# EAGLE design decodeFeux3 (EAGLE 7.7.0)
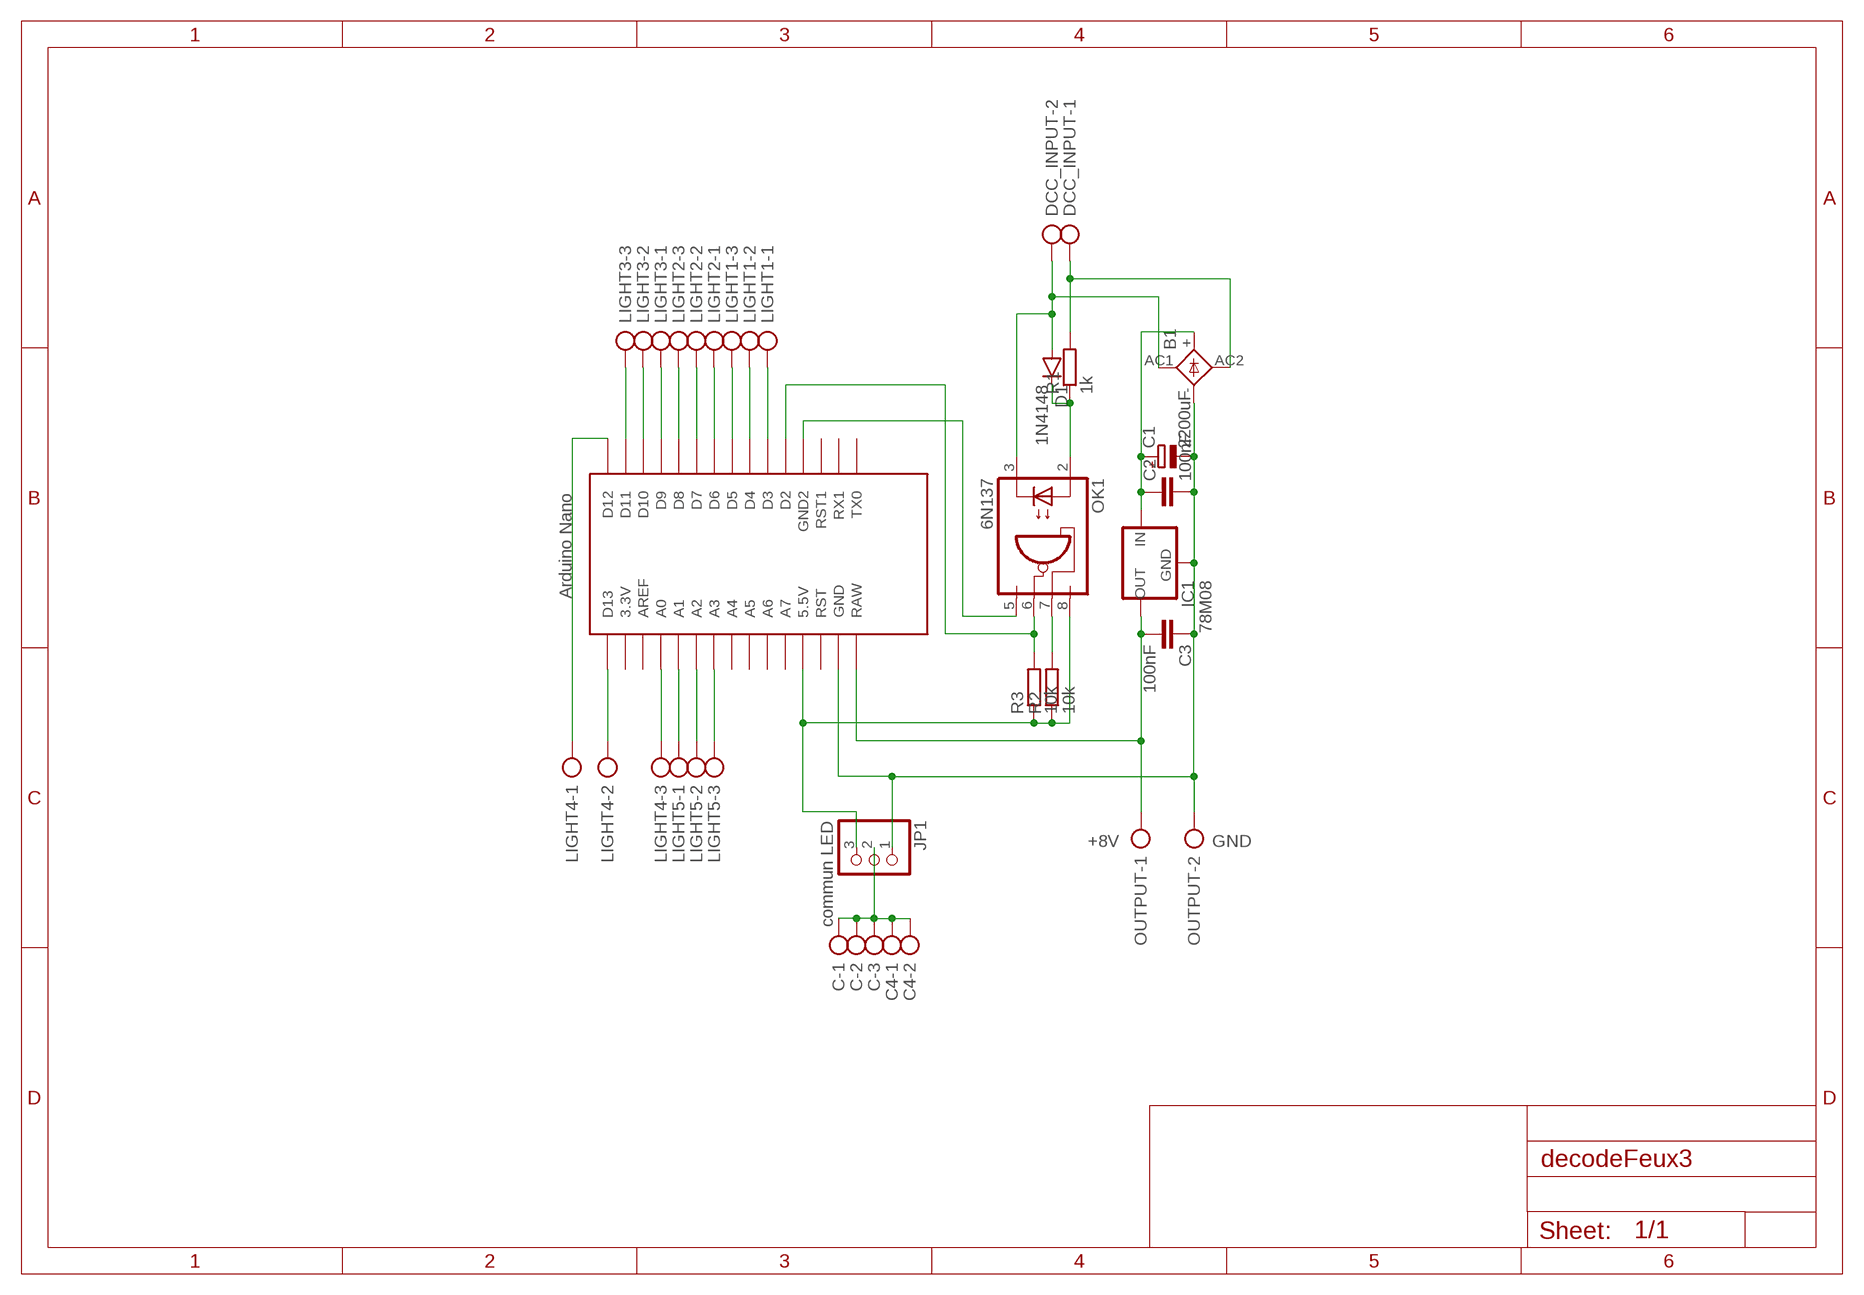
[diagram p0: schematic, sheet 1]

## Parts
B1  2KBP  [2KBP]
C  AK300/3  [AK300/3]
C1  2200uF  CPOL-EUE7.5-16  [E7,5-16]
C2  100nF  C-EU050-025X075  [C050-025X075]
C3  100nF  C-EU050-025X075  [C050-025X075]
C4  AK300/2  [AK300/2]
D1  1N4148  DIODE1N4148  [DIODE-1N4148]
DCC_INPUT  AK300/2  [AK300/2]
IC1  78M08  R-78C1.8-1.0  [SIP3]
JP1  commun LED  PINHD-1X3  [1X03]
LIGHT1  AK300/3  [AK300/3]
LIGHT2  AK300/3  [AK300/3]
LIGHT3  AK300/3  [AK300/3]
LIGHT4  AK300/3  [AK300/3]
LIGHT5  AK300/3  [AK300/3]
OK1  6N137  [DIL08]
OUTPUT  AK300/2  [AK300/2]
R1  1k  R-EU_0207/10  [0207/10]
R2  10k  R-EU_0207/10  [0207/10]
R3  10k  R-EU_0207/10  [0207/10]
U$1  NANO  [NANO]

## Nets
N$1: LIGHT4.1 U$1.D12
N$2: LIGHT3.3 U$1.D11
N$3: LIGHT3.2 U$1.D10
N$4: LIGHT3.1 U$1.D9
N$5: LIGHT2.3 U$1.D8
N$6: LIGHT2.2 U$1.D7
N$7: LIGHT2.1 U$1.D6
N$8: LIGHT1.3 U$1.D5
N$9: LIGHT1.2 U$1.D4
N$10: LIGHT1.1 U$1.D3
N$11: LIGHT4.2 U$1.D13
N$12: LIGHT4.3 U$1.A0
N$13: LIGHT5.1 U$1.A1
N$14: LIGHT5.2 U$1.A2
N$15: LIGHT5.3 U$1.A3
N$17: OK1.6(VO) R3.2 U$1.D2
N$18: OK1.7(VE) R2.2
N$19: JP1.3 OK1.8(VCC) R2.1 R3.1 U$1.5V(5.5V)
N$20: OK1.5(GND) U$1.GND1(GND2)
N$21: B1.AC2 DCC_INPUT.1 R1.2
N$22: B1.AC1 D1.A DCC_INPUT.2 OK1.3(C)
N$23: D1.C OK1.2(A) R1.1
N$24: B1.+ C1.+ C2.1 IC1.1(IN)
N$25: B1.- C1.- C2.2 C3.1 IC1.2(GND) JP1.1 OUTPUT.2 U$1.GND
N$26: C3.2 IC1.3(OUT) OUTPUT.1 U$1.RAW
N$28: C4.1 C4.2 C.1 C.2 C.3 JP1.2
Unconnected: U$1.3.3V U$1.A4 U$1.A5 U$1.A6 U$1.A7 U$1.AREF U$1.ICSP1 U$1.ICSP2 U$1.ICSP3 U$1.ICSP4 U$1.ICSP5 U$1.ICSP6 U$1.RST U$1.RST1 U$1.RX1 U$1.TX0

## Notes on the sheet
- +8V | GND

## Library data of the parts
B1 = rectifier:2KBP: RECTIFIER grid 3 x 3,81 mm
C LIGHT1-LIGHT5 = con-ptr500:AK300/3: CONNECTOR; OC_FARNELL: unknown; OC_NEWARK: unknown
C1 = resistor:CPOL-EU: POLARIZED CAPACITOR, European symbol
C2 C3 = rcl:C-EU: CAPACITOR, European symbol
C4 DCC_INPUT OUTPUT = con-ptr500:AK300/2: CONNECTOR; OC_FARNELL: unknown; OC_NEWARK: unknown
D1 = SparkFun-DiscreteSemi:DIODE: Diode; PROD_ID: DIO-08378
IC1 = r-78xx_10:R-78C*-1.0: Innoline R-78Cxx-1.0 Series Switching Regulators - 1.0A, Wide Input Range, High Efficiency Source: http://www.recom-international.com/pdf/Innoline/R-78Cxx-1.0.pdf; MF: Recom; MPN: R-78C1.8-1.0; OC_FARNELL: 1903038; OC_NEWARK: 62X9492
JP1 = adafruit:PINHD-1X3: PIN HEADER
OK1 = optocoupler:6N137: MOTOROLA OPTO COUPLER; MPN: 6N137; OC_FARNELL: 1328376; OC_NEWARK: 52M1895
R1-R3 = resistor:R-EU_: RESISTOR, European symbol
U$1 = Arduino-clone:NANO: Arduino Nano

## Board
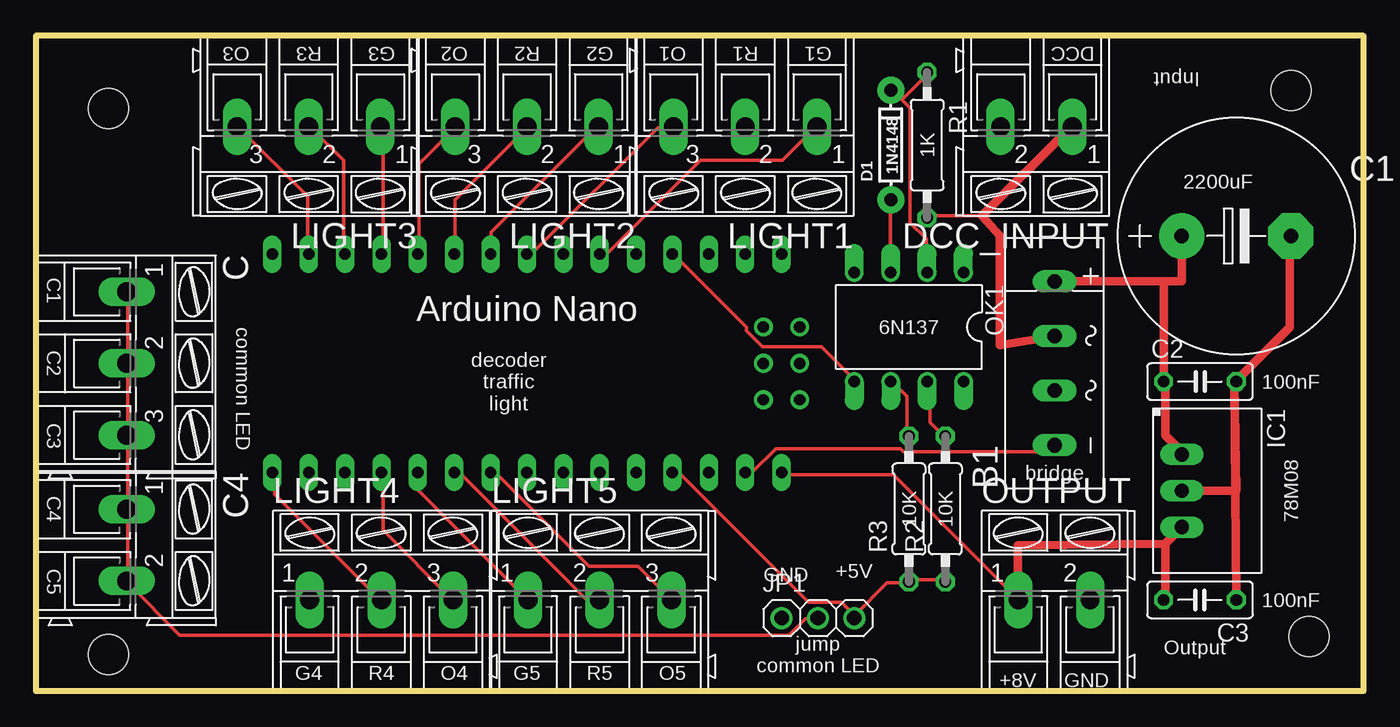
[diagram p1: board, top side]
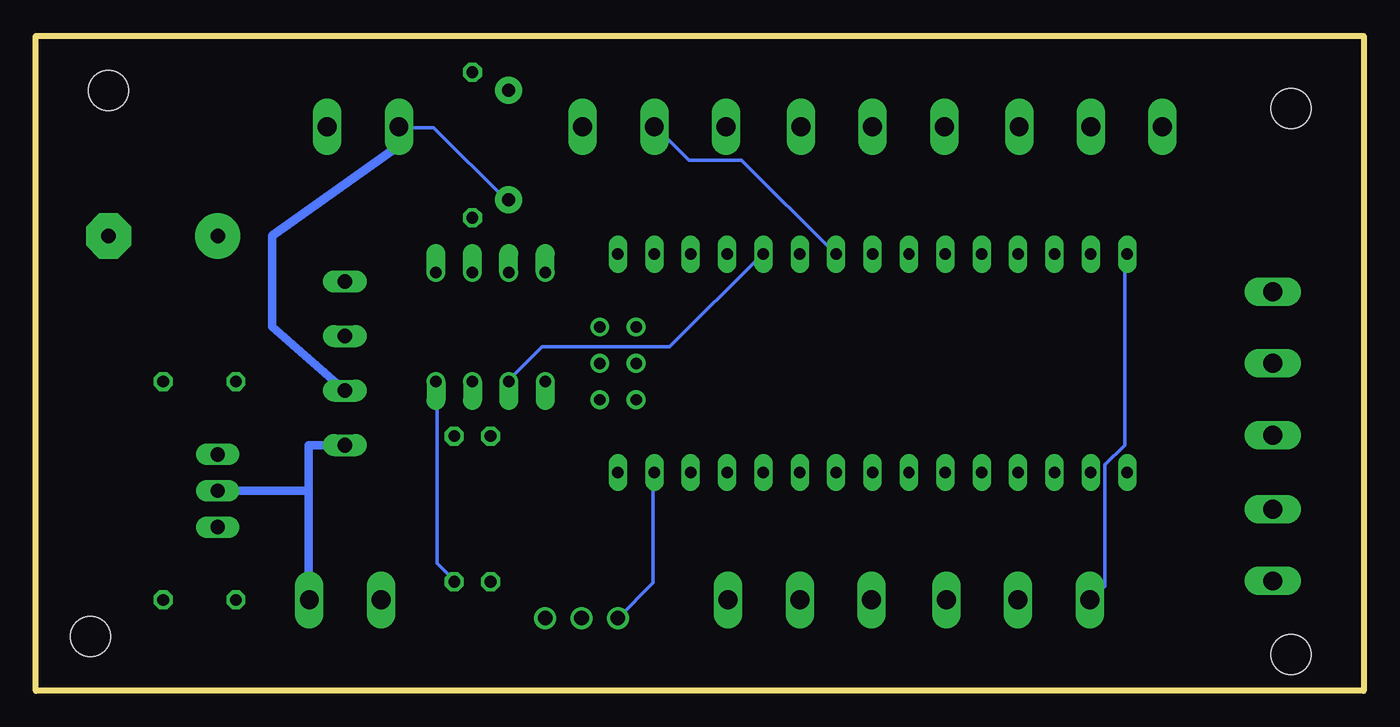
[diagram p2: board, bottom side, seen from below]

Size 92.71 x 45.72 mm. Coordinates in mm from the lower left corner, seen from the top.
Outline: 0,0 92.71,0 92.71,45.72 0,45.72 0,0
Copper layers (1*16): Top 0.035mm / dielectric 1.5mm / Bottom 0.035mm
Design rules "default": minimum track width 10mil, minimum drill 24mil, track to track 8mil, track to pad 8mil, pad to pad 8mil, via to via 8mil, smd to smd 8mil, copper to edge 40mil, drill to drill 8mil, minimum pad ring 10mil, minimum via ring 8mil, stop-mask expansion 4mil, vias tented up to drill 0mil, thermal gap 10mil
Holes 2.8 mm at 5.08,40.64 5.08,2.54 88.9,3.81 87.63,41.91

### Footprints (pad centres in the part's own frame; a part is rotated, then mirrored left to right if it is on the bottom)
2KBP = drill 1.016 long: + 5.715,0; - -5.715,0; AC1 -1.905,0; AC2 1.905,0
AK300/3 = drill 1.321 long: 1 -5.004,0; 2 0,0; 3 5.004,0
E7,5-16 = drill 1.016 pad 3.15: + -3.81,0 | drill 1.016 pad 3.15 octagon: - 3.81,0
C050-025X075 = drill 0.813 octagon: 1 -2.54,0; 2 2.54,0
AK300/2 = drill 1.321 long: 1 -2.515,0; 2 2.489,0
DIODE-1N4148 = drill 0.9 pad 1.88: A -3.81,0; C 3.81,0
SIP3 = drill 1 long: 1 -2.54,0; 2 0,0; 3 2.54,0
1X03 = drill 1.016: 1 -2.54,0; 2 0,0; 3 2.54,0
DIL08 = drill 0.813 offset: 1 -3.81,-3.81; 2 -1.27,-3.81; 3 1.27,-3.81; 4 3.81,-3.81; 5 3.81,3.81; 6 1.27,3.81; 7 -1.27,3.81; 8 -3.81,3.81
0207/10 = drill 0.813 octagon: 1 -5.08,0; 2 5.08,0
NANO = drill 0.8 long: 3.3V -10.16,24.13; 5V -10.16,-1.27; A0 -10.16,19.05; A1 -10.16,16.51; A2 -10.16,13.97; A3 -10.16,11.43; A4 -10.16,8.89; A5 -10.16,6.35; A6 -10.16,3.81; A7 -10.16,1.27; AREF -10.16,21.59; D2 5.08,1.27; D3 5.08,3.81; D4 5.08,6.35; D5 5.08,8.89; D6 5.08,11.43; D7 5.08,13.97; D8 5.08,16.51; D9 5.08,19.05; D10 5.08,21.59; D11 5.08,24.13; D12 5.08,26.67; D13 -10.16,26.67; GND -10.16,-6.35; GND1 5.08,-1.27; RAW -10.16,-8.89; RST -10.16,-3.81; RST1 5.08,-3.81; RX1 5.08,-6.35; TX0 5.08,-8.89 | drill 0.8: ICSP1 -5.08,-10.16; ICSP2 -5.08,-7.62; ICSP3 -2.54,-10.16; ICSP4 -2.54,-7.62; ICSP5 0,-10.16; ICSP6 0,-7.62

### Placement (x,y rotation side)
B1  71.12,22.86 90 top
C  6.35,22.86 270 top
C1  83.82,31.75 0 top
C2  81.28,21.59 0 top
C3  81.28,6.35 180 top
C4  6.35,10.16 270 top
D1  59.69,38.1 90 top
DCC_INPUT  69.85,39.37 180 top
IC1  80.01,13.97 270 top
JP1  54.61,5.08 0 top
LIGHT1  49.53,39.37 180 top
LIGHT2  34.29,39.37 180 top
LIGHT3  19.05,39.37 180 top
LIGHT4  24.13,6.35 0 top
LIGHT5  39.37,6.35 0 top
OK1  60.96,25.4 180 top
OUTPUT  71.12,6.35 0 top
R1  62.23,38.1 270 top
R2  63.5,12.7 90 top
R3  60.96,12.7 90 top
U$1  43.18,25.4 90 top

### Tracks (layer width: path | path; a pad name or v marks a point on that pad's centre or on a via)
N$1
  Bottom 0.254: U$1.D12 16.69,30.4 16.69,17.14 18.06,15.77 18.06,7.32 18.97,6.4 LIGHT4.1
N$2
  Top 0.254: U$1.D11 18.97,30.63 18.97,34.52 14.17,39.32 LIGHT3.3
N$3
  Top 0.254: U$1.D10 21.49,30.63 21.49,37.03 19.2,39.32 LIGHT3.2
N$4
  Top 0.254: U$1.D9 24.23,30.63 24.23,39.32 LIGHT3.1
N$5
  Top 0.254: U$1.D8 26.75,30.63 26.75,36.8 29.26,39.32 LIGHT2.3
N$6
  Top 0.254: U$1.D7 29.26,30.63 29.26,34.29 34.29,39.32 LIGHT2.2
N$7
  Top 0.254: U$1.D6 31.77,30.63 31.77,32 39.09,39.32 LIGHT2.1
N$8
  Top 0.254: U$1.D5 34.29,30.63 34.75,30.63 43.43,39.32 44.35,39.32 LIGHT1.3
N$9
  Bottom 0.254: U$1.D4 37.03,30.63 43.43,37.03 47.09,37.03 49.38,39.32 LIGHT1.2
N$10
  Top 0.254: U$1.D3 39.55,30.63 40.01,30.63 46.41,37.03 52.12,37.03 54.41,39.32 LIGHT1.1
N$11
  Top 0.254: U$1.D13 16.69,15.09 16.69,13.72 24,6.4 LIGHT4.2
N$12
  Top 0.254: U$1.A0 24.23,15.09 24.23,11.2 29.03,6.4 LIGHT4.3
N$13
  Top 0.254: U$1.A1 26.75,15.09 26.75,13.95 34.29,6.4 LIGHT5.1
N$14
  Top 0.254: U$1.A2 29.26,15.09 29.72,15.09 38.41,6.4 39.32,6.4 LIGHT5.2
N$15
  Top 0.254: U$1.A3 31.77,15.09 32.23,15.09 38.63,8.69 42.06,8.69 44.35,6.4 LIGHT5.3
N$17
  Top 0.254: R3.2 60.81,17.83 60.81,20.57 59.89,21.49 OK1.6
  Bottom 0.254: U$1.D2 42.06,30.4 48.46,24 57.38,24 59.66,21.72 OK1.6
N$18
  Top 0.254: OK1.7 62.41,21.49 62.41,18.75 63.32,17.83 R2.2
N$19
  Top 0.254: R2.1 63.32,7.77 61.04,7.77 R3.1 60.81,7.54 59.44,7.54 57.15,5.26 | 57.15,5.26 56.24,6.17 53.95,6.17 45.03,15.09 44.58,15.09 U$1.5V | 57.15,5.26 JP1.3
  Bottom 0.254: OK1.8 64.69,21.49 64.69,8.91 63.55,7.77 R2.1
N$20
  Top 0.254: U$1.GND1 44.58,30.4 49.61,25.38 49.61,25.15 50.75,24 54.86,24 57.15,21.72 OK1.5
N$21
  Top 0.254: 66.06,33.15 62.41,33.15 R1.2 | 72.24,39.32 DCC_INPUT.1 | 71.09,24.92 B1.AC2
  Top 0.61: 72.24,39.32 66.06,33.15 67.31,31.75 67.31,24.13 B1.AC2
N$22
  Top 0.254: D1.A 59.66,34.29 59.66,29.26 OK1.3 59.89,29.03
  Bottom 0.254: DCC_INPUT.2 67.21,39.32 64.92,39.32 59.89,34.29 D1.A
  Bottom 0.61: B1.AC1 76.2,25.4 76.2,31.75 67.31,38.1 DCC_INPUT.2
N$23
  Top 0.254: 60.35,41.38 59.89,41.83 D1.C 60.35,41.38 | 60.35,41.38 61.04,40.69 61.04,32.69 62.18,31.55 62.18,29.26 OK1.2 | 60.35,41.38 60.58,41.38 62.18,42.98 R1.1
N$24
  Top 0.254: 78.87,21.49 C2.1 | 80.01,16.69 IC1.1
  Top 0.61: 78.87,21.49 78.87,17.83 80.01,16.69 | B1.+ 78.74,28.57 | 78.74,28.57 80.01,28.57 C1.+ | C2.1 78.74,28.57
N$25
  Top 0.254: 80.01,13.95 IC1.2 80.01,14.17 | 83.67,21.49 C2.2 83.9,21.72 | 87.55,31.55 C1.- | U$1.GND 49.61,15.32 50.06,15.32 51.66,16.92 60.35,16.92 60.58,16.69 70.64,16.69 71.09,17.14 B1.-
  Top 0.61: 87.55,31.55 87.55,25.38 83.9,21.72 | C3.1 83.67,21.49 83.82,13.97 IC1.2
  Bottom 0.254: JP1.1 49.61,7.54 49.61,15.09 U$1.GND | 80.01,13.95 IC1.2 | OUTPUT.2 73.61,6.4 73.66,6.4
  Bottom 0.61: 73.66,13.97 73.66,6.4 73.66,6.35 | B1.- 73.66,17.14 73.66,13.97 | 73.66,13.97 IC1.2
N$26
  Top 0.254: 78.87,6.4 C3.2 | U$1.RAW 52.12,15.09 59.89,15.09 68.58,6.4 OUTPUT.1 68.81,6.4
  Top 0.61: 78.87,10.29 78.87,6.4 | IC1.3 78.87,10.29 | 78.87,10.29 68.58,10.16 OUTPUT.1
N$28
  Top 0.254: 6.4,22.86 6.4,18.06 C.3 6.4,17.83 6.4,12.8 C4.1 6.4,12.57 6.4,7.77 C4.2 6.4,7.54 10.06,3.89 52.58,3.89 53.72,5.03 54.41,5.03 JP1.2 | 6.4,22.86 6.4,27.66 C.1 | 6.4,22.86 C.2

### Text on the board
tPlace: O3 | R3 | G3 | O2 | R2 | G2 | O1 | R1 | G1 | DCC | Input | 1K | 2200uF | C1 | Arduino Nano | common LED | 6N137 | C2 | decoder / traffic / light | 100nF | C3 | bridge | 78M08 | C4 | 10K | 10K | +5V | C5 | GND | 100nF | jump / common LED | Output | G4 | R4 | O4 | G5 | R5 | O5 | +8V | GND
